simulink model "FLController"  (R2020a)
settings: Solver=VariableStepAuto  StartTime=0.0  StopTime=10.0  RelTol=1e-3
InitFcn:
  | initParams
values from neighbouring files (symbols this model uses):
  K1 = 5    [initParams.m]
  K2 = 10    [initParams.m]
  K3 = 50    [initParams.m]
  x0 = [0.2;0.1]    [initParams.m]

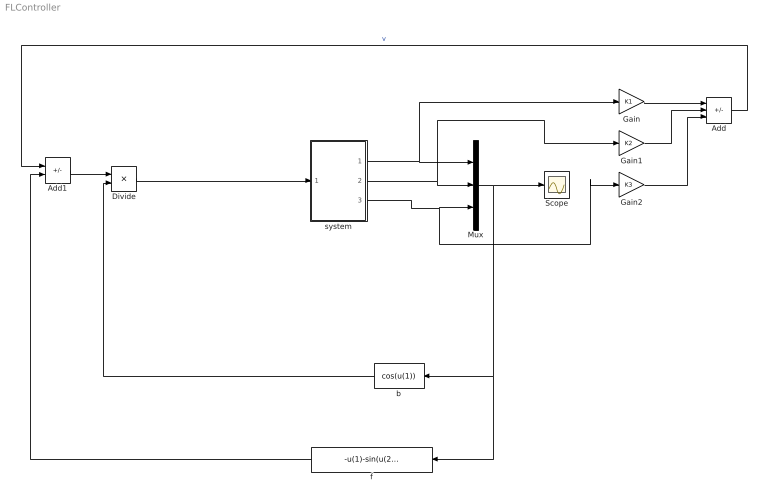
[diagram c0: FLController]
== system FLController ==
  Add : Sum  Inputs=---
  Add1 : Sum  Inputs=+-
  Divide : Product  Inputs=*/
  Gain : Gain  Gain=K1
  Gain1 : Gain  Gain=K2
  Gain2 : Gain  Gain=K3
  Mux : Mux  Inputs=3
  Scope : Scope
  b : Fcn  Expr=cos(u(1))
  f : Fcn  Expr=-u(1)-sin(u(2))-sin(u(3))
  system : Subsystem
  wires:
  system/1(x1) -> Gain/1, Mux/1
  system/2(x2) -> Mux/2, Gain1/1
  system/3(x3) -> Gain2/1, Mux/3
  Mux/1 -> Scope/1, f/1, b/1
  Gain/1 -> Add/1
  Gain1/1 -> Add/2
  Add/1 -> Add1/1  "v"
  f/1 -> Add1/2
  Add1/1 -> Divide/1
  b/1 -> Divide/2
  Divide/1 -> system/1(u)
  Gain2/1 -> Add/3

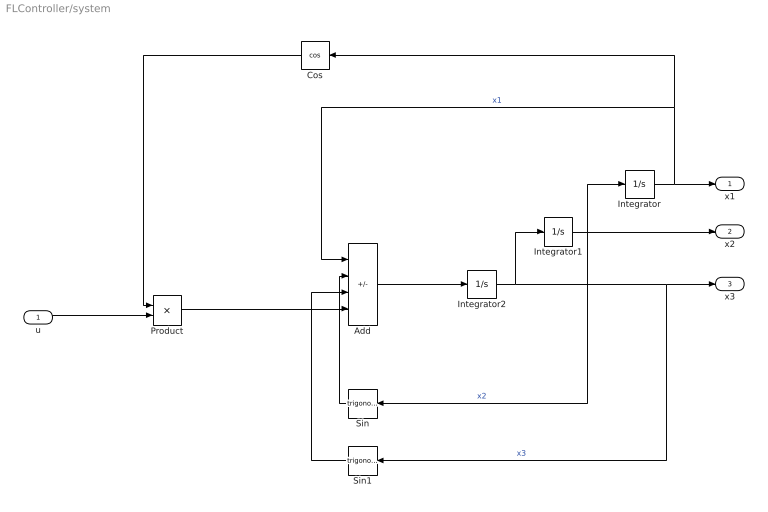
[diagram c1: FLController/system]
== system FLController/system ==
  u : Inport
  Add : Sum  Inputs=---+
  Cos : Trigonometry  Operator=cos
  Integrator : Integrator  InitialCondition=x0(1)
  Integrator1 : Integrator  InitialCondition=x0(2)
  Integrator2 : Integrator  InitialCondition=x0(3)
  Product : Product
  Sin : Trigonometry
  Sin1 : Trigonometry
  x1 : Outport
  x2 : Outport  Port=2
  x3 : Outport  Port=3
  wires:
  Integrator1/1 -> x2/1, Sin/1, Integrator/1  "x2"
  Product/1 -> Add/4
  Integrator2/1 -> x3/1, Sin1/1, Integrator1/1  "x3"
  Integrator/1 -> x1/1, Add/1, Cos/1  "x1"
  Add/1 -> Integrator2/1
  u/1 -> Product/2
  Cos/1 -> Product/1
  Sin1/1 -> Add/3
  Sin/1 -> Add/2
